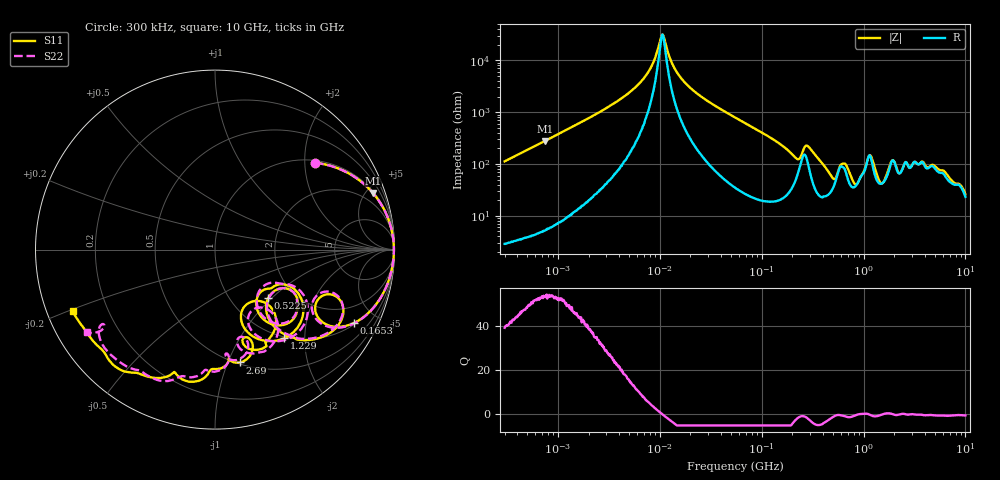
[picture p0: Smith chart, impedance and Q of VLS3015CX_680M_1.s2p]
! S-Parameter Data Generated by TDK Corporation
! Copyright(C) 2020 TDK Corporation.
! All Rights Reserved.
! TDK P/N: VLS3015CX-680M-1 (Inductor)
! Property: L=68uH at 1MHz
! Size(LxWxT): 3x3x1.5mm
! Model Type: s2p (Touchstone File Format Version 1.0)
! Frequency: DC=Yes Start=0.3MHz Stop=10000MHz 802points Log-sweep
! Model Generated on Aug. 18, 2020
! Port Assignments:
!  1 ---@@@--- 2
! Applicable Conditions:
!  Temperature = 25 degC
!  DC Bias Current = 0 A
!  Small Signal Operation
! Terms and conditions regarding TDK Simulation Models
! (1)This simulation model is being provided solely for informational purposes. Please refer to the specifications of the products in terms of detailed characteristics of such products.
! (2)In no event shall TDK Corporation of any of its subsidiaries be liable for any loss or damage arising, directly or indirectly,
!  From any information contained in this simulation model, including, but not limited to loss or damages arising from any inaccuracies, omissions or errors in connection with such information.
! (3)Any and all copyrights on this simulation model are owned by TDK Corporation.
!  Duplication or redistribution of this simulation model without prior written permission from TDK Corporation is prohibited.
! (4)This simulation model is subject to any modification or change without any prior notice.
! (5)Neither TDK Corporation nor any of its subsidiaries shall make any warranty, express or implied,
!  Including but not limited to the correctness, implied warranties of merchantability and fitness for a particular purpose with respect to this simulation models.
! (6)The use of this simulation model shall be deemed to have consented to the terms and conditions hereof.
# Hz S MA R 50
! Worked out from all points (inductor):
!   801 points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, 300 kHz to 10 GHz, reference 50 ohm
!   read as one part in series: L = 59.5 uH near 318.3 kHz
!   highest Q = 53.3 at 742.2 kHz (marker M1), where L = 59.5 uH
!   self-resonance near 10.62 MHz
!   S11 on the Smith chart (normalised r, x): 300 kHz: 1.06, +2.25; 165.3 MHz: 1.07, -3.77; 522.5 MHz: 1.47, -0.95; 1.229 GHz: 0.98, -1.59; 2.69 GHz: 0.52, -1.11; 10 GHz: 0.08, -0.21
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300000  0.7383 41.0  0.656 -47.5  0.6559 -47.5  0.7377 41.0
742172  0.9347 19.7  0.337 -69.2  0.3369 -69.2  0.9348 19.7
1713600  0.9847 8.7  0.1514 -79.9  0.1514 -80.0  0.9849 8.7
5955893  0.9966 1.6  0.03101 -83.3  0.03107 -83.1  0.9967 1.6
9671944  0.9968 0.0  0.005708 -56.9  0.005721 -56.9  0.9969 -0.0
1.07612e7  0.9967 -0.3  0.003227 10.0  0.003217 10.1  0.9967 -0.3
1.35567e7  0.9966 -1.1  0.0127 73.9  0.0127 74.0  0.9966 -1.1
1.740512e7  0.9962 -1.9  0.02587 80.5  0.02587 80.5  0.9962 -2.0
5.477226e7  0.9867 -8.6  0.1241 78.9  0.124 78.9  0.9867 -8.6
1.653189e8  0.8768 -27.7  0.4003 56.2  0.4002 56.2  0.8751 -28.1
2.53844e8  0.69 -21.2  0.3763 18.9  0.3762 18.9  0.6717 -20.4
3.126428e8  0.8019 -33.3  0.428 42.2  0.4279 42.1  0.7977 -32.4
4.089972e8  0.6495 -48.7  0.6238 28.4  0.6236 28.4  0.6493 -48.1
5.225392e8  0.4014 -42.5  0.6711 2.6  0.6709 2.6  0.404 -42.0
7.152593e8  0.5442 -50.8  0.6013 8.7  0.6012 8.7  0.5414 -49.6
9.903836e8  0.3872 -31.9  0.589 -24.3  0.5888 -24.3  0.4224 -26.9
1.228555e9  0.6272 -51.9  0.4391 -5.5  0.4389 -5.5  0.6442 -50.3
1.459486e9  0.4301 -69.8  0.6384 -19.4  0.638 -19.4  0.4585 -65.9
1.767019e9  0.418 -46.2  0.5307 -46.6  0.5304 -46.6  0.4857 -47.9
2.69003e9  0.6442 -77.5  0.3804 -48.2  0.3804 -48.2  0.625 -80.6
6.091595e9  0.8327 -124.8  0.2342 -71.0  0.2339 -71.2  0.8062 -124.3
1e10  0.8637 -156.6  0.1898 -82.8  0.1892 -82.8  0.8478 -147.0
